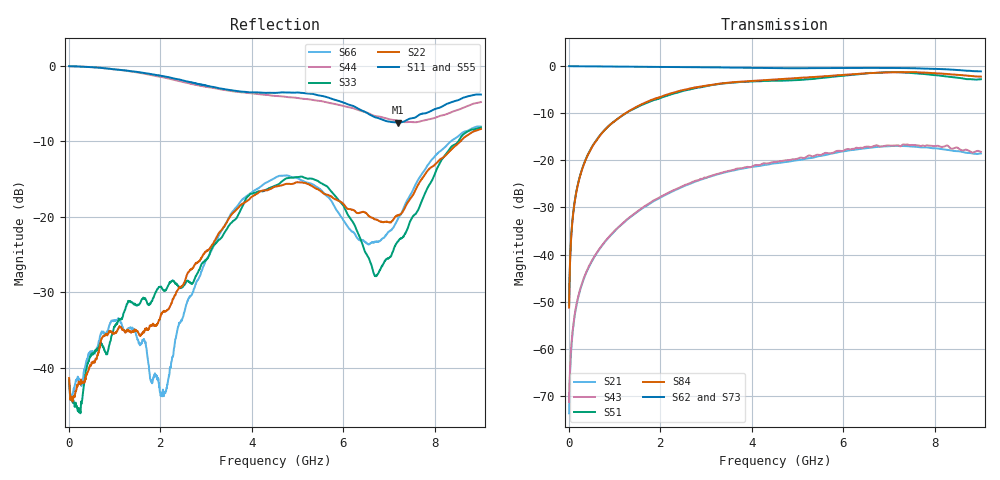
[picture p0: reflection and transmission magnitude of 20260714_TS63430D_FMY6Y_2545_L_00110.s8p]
# GHz S DB R 50
! CMT, SN0916, 25263762, 26.7.0
! Date: 15.07.2026 14:54:46
! Data: Format
! Freq S1.1:dB/Ang S1.2:dB/Ang S1.3:dB/Ang S1.4:dB/Ang S1.5:dB/Ang S1.6:dB/Ang S1.7:dB/Ang S1.8:dB/Ang
!  S2.1:dB/Ang S2.2:dB/Ang S2.3:dB/Ang S2.4:dB/Ang S2.5:dB/Ang S2.6:dB/Ang S2.7:dB/Ang S2.8:dB/Ang
!  S3.1:dB/Ang S3.2:dB/Ang S3.3:dB/Ang S3.4:dB/Ang S3.5:dB/Ang S3.6:dB/Ang S3.7:dB/Ang S3.8:dB/Ang
!  S4.1:dB/Ang S4.2:dB/Ang S4.3:dB/Ang S4.4:dB/Ang S4.5:dB/Ang S4.6:dB/Ang S4.7:dB/Ang S4.8:dB/Ang
!  S5.1:dB/Ang S5.2:dB/Ang S5.3:dB/Ang S5.4:dB/Ang S5.5:dB/Ang S5.6:dB/Ang S5.7:dB/Ang S5.8:dB/Ang
!  S6.1:dB/Ang S6.2:dB/Ang S6.3:dB/Ang S6.4:dB/Ang S6.5:dB/Ang S6.6:dB/Ang S6.7:dB/Ang S6.8:dB/Ang
!  S7.1:dB/Ang S7.2:dB/Ang S7.3:dB/Ang S7.4:dB/Ang S7.5:dB/Ang S7.6:dB/Ang S7.7:dB/Ang S7.8:dB/Ang
!  S8.1:dB/Ang S8.2:dB/Ang S8.3:dB/Ang S8.4:dB/Ang S8.5:dB/Ang S8.6:dB/Ang S8.7:dB/Ang S8.8:dB/Ang
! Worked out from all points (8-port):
!   2001 points, 10 MHz to 9 GHz, reference 50 ohm
!   strongest paths, dB at 10 MHz, 2.257 GHz, 4.505 GHz, 6.753 GHz, 9 GHz:
!     S62: -0.1, -0.3, -0.5, -0.4, -1.2
!     S73: -0.1, -0.3, -0.5, -0.5, -1.2
!     S84: -51.2, -5.8, -2.9, -1.5, -2.3
!     S51: -50.8, -6.0, -3.1, -1.5, -2.8
!     S43: -71.2, -26.5, -20.4, -16.9, -18.2
!     S21: -73.6, -26.7, -20.7, -17.2, -18.6
!   lowest |S11| = -7.5 dB at 7.18 GHz (marker M1), VSWR 2.46, Z = 21.2 - j9.53 ohm
!   |S11| at or under -10 dB: nowhere
